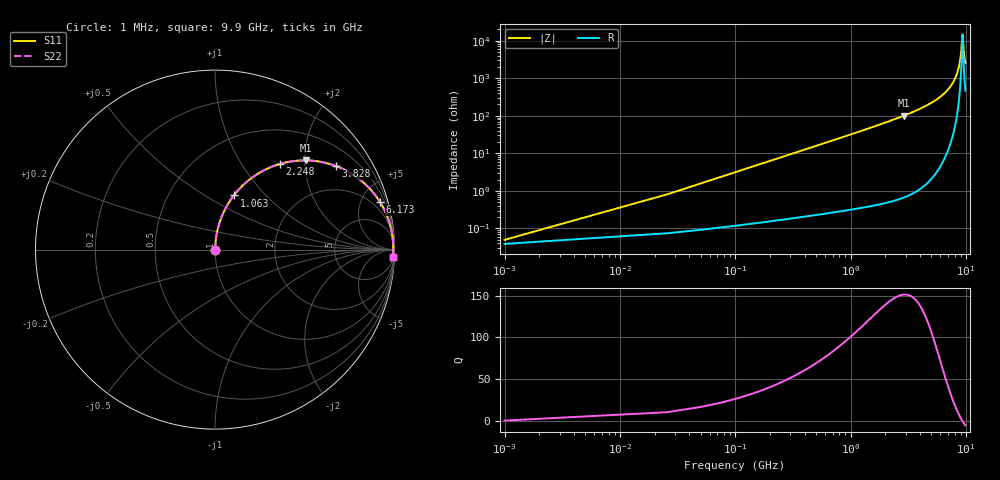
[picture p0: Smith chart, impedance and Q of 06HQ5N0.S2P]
! Coilcraft 0604HQ-5N0 Chip Inductor
! 15 August 2002
# MHZ S MA R 50
!Freq  MagS11  AngS11  MagS21  AngS21  MagS12  AngS12  MagS22  AngS22
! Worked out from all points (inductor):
!   402 points, 1 MHz to 9.9 GHz, reference 50 ohm
!   read as one part in series: L = 5 nH near 50.38 MHz
!   highest Q = 151 at 2.914 GHz (marker M1), where L = 5.54 nH
!   self-resonance near 9.334 GHz
!   S11 on the Smith chart (normalised r, x): 1 MHz: 1.00, +0.00; 1.063 GHz: 1.01, +0.68; 2.248 GHz: 1.01, +1.50; 3.828 GHz: 1.02, +2.89; 6.173 GHz: 1.10, +6.88; 9.9 GHz: 10, -49
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1  0.000499 39.0  0.9996 -0.0  0.9996 -0.0  0.000499 39.0
75.07  0.02358 86.1  0.9987 -1.3  0.9987 -1.3  0.02358 86.1
124.45  0.03905 85.9  0.998 -2.2  0.998 -2.2  0.03905 85.9
198.52  0.0622 85.0  0.9965 -3.6  0.9965 -3.6  0.0622 85.0
321.97  0.1006 83.2  0.9931 -5.8  0.9931 -5.8  0.1006 83.2
519.49  0.1612 79.9  0.9846 -9.3  0.9846 -9.3  0.1612 79.9
1062.67  0.3195 70.8  0.9445 -18.6  0.9445 -18.6  0.3195 70.8
1655.23  0.4715 61.4  0.8782 -28.1  0.8782 -28.1  0.4715 61.4
2247.79  0.5978 52.9  0.7975 -36.7  0.7975 -36.7  0.5978 52.9
2914.42  0.7097 44.4  0.6998 -45.2  0.6998 -45.2  0.7097 44.4
3309.46  0.7627 39.9  0.6416 -49.7  0.6416 -49.7  0.7627 39.9
3827.95  0.8196 34.6  0.5672 -55.0  0.5672 -55.0  0.8196 34.6
4963.69  0.9052 24.6  0.4168 -64.8  0.4168 -64.8  0.9052 24.6
6173.5  0.9564 16.1  0.278 -73.0  0.278 -73.0  0.9564 16.1
6617.92  0.9682 13.4  0.2323 -75.5  0.2323 -75.5  0.9682 13.4
8272.15  0.9909 4.7  0.08284 -81.3  0.08284 -81.3  0.9909 4.7
8914.09  0.9932 1.8  0.03271 -77.1  0.03271 -77.1  0.9932 1.8
9086.92  0.9933 1.1  0.02017 -70.2  0.02017 -70.2  0.9933 1.1
9333.82  0.9933 0.1  0.006796 -8.1  0.006796 -8.1  0.9933 0.1
9407.89  0.9932 -0.3  0.008091 32.5  0.008091 32.5  0.9932 -0.3
9654.79  0.9927 -1.3  0.023 70.8  0.023 70.8  0.9927 -1.3
9900  0.9919 -2.2  0.03951 77.1  0.03951 77.1  0.9919 -2.2
